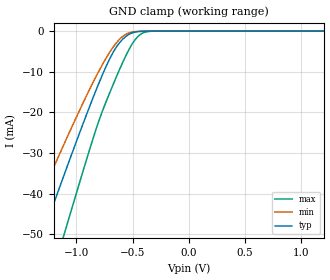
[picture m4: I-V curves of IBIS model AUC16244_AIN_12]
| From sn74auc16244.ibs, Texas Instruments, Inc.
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[Model]   AUC16244_AIN_12
Model_type  Input
Vinl=0.385
Vinh=0.845
| variable   typ   min   max
C_comp   3.30pF   2.74pF   3.82pF
[Temperature Range]   40   100   -40
| Ambient temperature   25   85   -40
[Voltage range]   1.2   1.1   1.3
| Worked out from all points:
|   GND clamp passes 1 mA (typ) near -0.54 V on its own axis
[GND Clamp]
| AUC16244_AIN_12
|   Voltage   I(typ)   I(min)   I(max)
-3.6V     -231.9mA   -193.8mA   -279.4mA
-1.46V    -62.59mA   -49.99mA   -82.84mA
-1.415V   -59.07mA   -47.09mA   -78.65mA
-1.285V   -48.96mA   -38.8mA    -66.53mA
-1.12V    -36.28mA   -28.5mA    -51.14mA
-1.085V   -33.62mA   -26.35mA   -47.88mA
-830mV    -14.93mA   -11.49mA   -24.63mA
-690mV    -6.122mA   -4.655mA   -14.32mA
-570mV    -1.564mA   -967.3uA   -6.667mA
-440mV    -101.1uA   -47.98uA   -1.031mA
-320mV    -3.023uA   -1.854uA   -27.1uA
1.2V      143.9pA    240.2pA    132.8pA
